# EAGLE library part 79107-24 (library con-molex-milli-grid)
RECEPTACAL
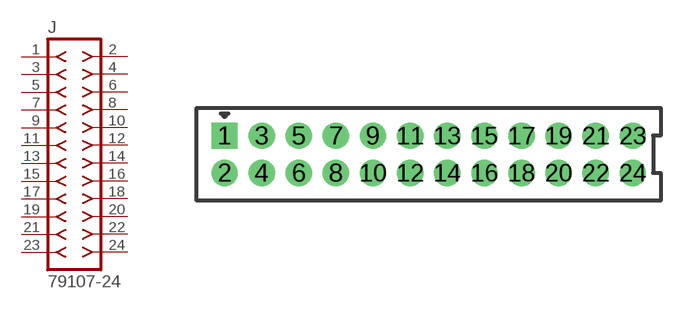
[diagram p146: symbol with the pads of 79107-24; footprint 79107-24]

Designator prefix J

## 79107-24  [79107-24]
1  1  pas
2  2  pas
3  3  pas
4  4  pas
5  5  pas
6  6  pas
7  7  pas
8  8  pas
9  9  pas
10  10  pas
11  11  pas
12  12  pas
13  13  pas
14  14  pas
15  15  pas
16  16  pas
17  17  pas
18  18  pas
19  19  pas
20  20  pas
21  21  pas
22  22  pas
23  23  pas
24  24  pas

## Footprint 79107-24 (pad centres in mm)
RECEPTACAL Dual Row, Vertical, Through-Hole
drill 0.914 square: 1 -11,1
drill 0.914: 2 -11,-1; 3 -9,1; 4 -9,-1; 5 -7,1; 6 -7,-1; 7 -5,1; 8 -5,-1; 9 -3,1; 10 -3,-1; 11 -1,1; 12 -1,-1; 13 1,1; 14 1,-1; 15 3,1; 16 3,-1; 17 5,1; 18 5,-1; 19 7,1; 20 7,-1; 21 9,1; 22 9,-1; 23 11,1; 24 11,-1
